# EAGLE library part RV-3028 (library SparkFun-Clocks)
RV-3028 - RTC with I2C Bus Specifications: Pin count: 8 Pin pitch: .9mm Area: [3.2mm x 2.0mm] Datasheet referenced for footprint
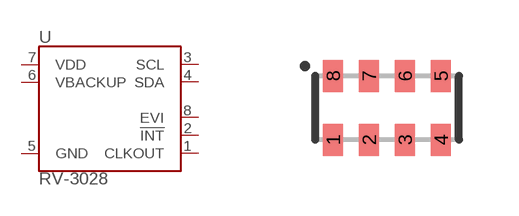
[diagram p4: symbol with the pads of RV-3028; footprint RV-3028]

Designator prefix U

## RV-3028 (PROD_ID: IC-14378)  [RV-3028]
1  CLKOUT
2  !INT
3  SCL
4  SDA
5  GND
6  VBACKUP
7  VDD
8  EVI

## Footprint RV-3028 (pad centres in mm)
Footprint for the RV-3028 I2C RTC
smd 0.5 x 0.8: 1 -1.35,-0.8; 2 -0.45,-0.8; 3 0.45,-0.8; 4 1.35,-0.8; 5 1.35,0.8; 6 0.45,0.8; 7 -0.45,0.8; 8 -1.35,0.8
